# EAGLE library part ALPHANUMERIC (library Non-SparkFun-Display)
Alphanumeric LED Display Common anode. Multiple LEDs on some segments. Multiple LED colors available. Works great with A6282 driver IC. Decimal points are unfornately not connected. SKU: COM-09933.
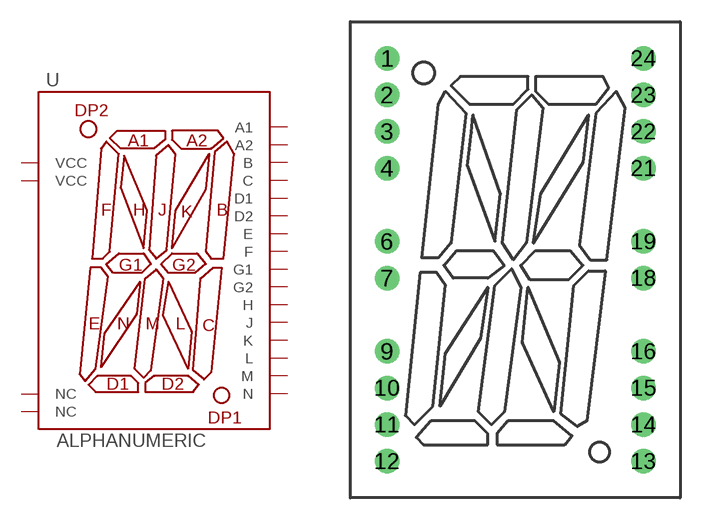
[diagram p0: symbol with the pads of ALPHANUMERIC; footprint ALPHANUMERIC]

Designator prefix U

## ALPHANUMERICPTH  [ALPHANUMERIC]
1  NC
2  A1
3  H
4  F
6  VCC
7  G1
9  E
10  D1
11  N
12  M
13  NC
14  D2
15  L
16  C
18  VCC
19  G2
21  B
22  A2
23  K
24  J

## Footprint ALPHANUMERIC (pad centres in mm)
drill 0.9 pad 1.7: 1 -8.89,13.97; 2 -8.89,11.43; 3 -8.89,8.89; 4 -8.89,6.35; 6 -8.89,1.27; 7 -8.89,-1.27; 9 -8.89,-6.35; 10 -8.89,-8.89; 11 -8.89,-11.43; 12 -8.89,-13.97; 13 8.89,-13.97; 14 8.89,-11.43; 15 8.89,-8.89; 16 8.89,-6.35; 18 8.89,-1.27; 19 8.89,1.27; 21 8.89,6.35; 22 8.89,8.89; 23 8.89,11.43; 24 8.89,13.97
